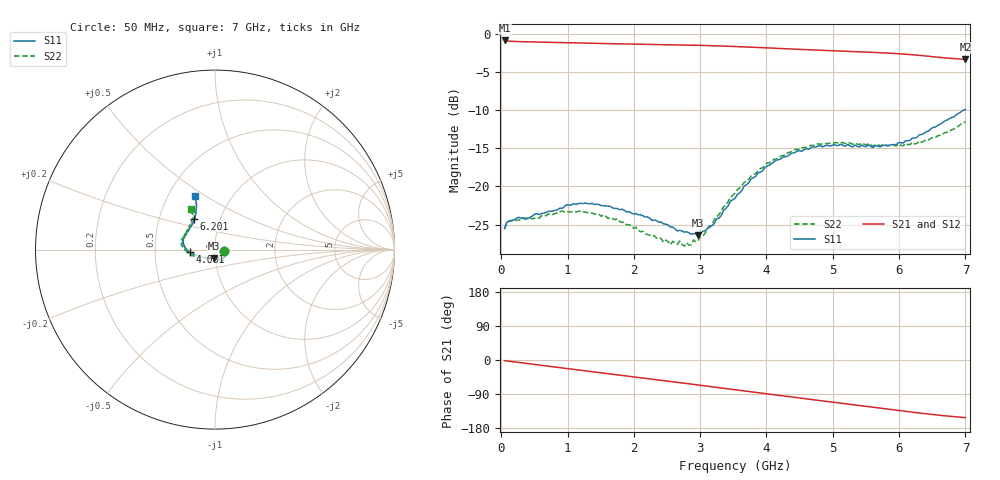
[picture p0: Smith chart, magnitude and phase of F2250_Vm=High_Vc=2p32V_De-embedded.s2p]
! Integrated Device Technology
! Corporate Headquarters
! 6024 Silver Creek Valley Road
! San Jose, CA 95138  USA
! Phone:  1-408-284-8200
! Toll Free:  1-800-223-1366
! Webpage:  http://www.idt.com/
! Timing and RF Division
! 515 Groton Road, Suite 102
! Westford, MA 01886-6024
! Device:  F2250
! Description: Voltage Variable RF Attenuator
! Frequency:  50.0 -  6000.00 MHz
! Package:  3x3 mm Thin QFN Plastic Package: 16 pin
! Ports:  2 RF, 3 DC
!  Pin  1  = GND
!  Pin  2  = NC
!  Pin  3  = RF1  = Port 1
!  Pin  4  = NC
!  Pin  5  = GND
!  Pin  6  = GND
!  Pin  7  = GND
!  Pin  8  = GND
!  Pin  9  = NC
!  Pin 10  = RF2  = Port 2
!  Pin 11  = NC
!  Pin 12  = GND
!  Pin 13  = GND
!  Pin 14  = VCNTRL
!  Pin 15  = VDD
!  Pin 16  = VMODE
! Vcntrl:  2.320 Volts
! Vmode:  +3.300 Volts
! Vdd:  +3.30  Volts
! Current:  1.314 mA
! Data:  The device was measured on a the F2250 evaluation board which has
!  individual transmission lines to the RF pins.  Data was collected
!  using a calibrated network analyzer.  The evaluation board was
!  de-embedded using a TRL calibration technique.
!  The reference plane is the edge of the package pin.
! Misc:  SN 10
!  Action Tracker AT0258
! Date Measured:  2014-11-26
! Date:  2015-10-15  MJV
! Note:
!  Integrated Device Technology supplies this data as a sample of measured
!  data at the package pin for this product.  Your particular data for this
!  product may vary.
!  Data was taken at 25 degrees C.
!  Integrated Device Technology reserves the right to change this data at anytime.
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# GHz S dB R 50
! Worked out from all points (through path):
!   201 points, 50 MHz to 7 GHz, reference 50 ohm
!   highest |S21| = -0.90 dB at 50 MHz (marker M1); lowest = -3.4 dB at 7 GHz (marker M2)
!   group delay of S21, straight-line fit = 61.2 ps
!   lowest |S11| = -26.3 dB at 2.969 GHz (marker M3), VSWR 1.10, Z = 49.2 - j4.73 ohm
!   |S11| at or under -10 dB: start of sweep to 6.978 GHz
!   |S22| runs from -27.8 to -11.5 dB; largest |S21 - S12| = 0.0019
!   S11 on the Smith chart (normalised r, x): 50 MHz: 1.11, -0.02; 4.081 GHz: 0.75, -0.02; 6.201 GHz: 0.75, +0.27; 7 GHz: 0.68, +0.45
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0.05  -25.45 -10.4  -0.90 -1.8  -0.90 -1.8  -25.61 -10.7
0.1195  -24.55 -10.0  -1.00 -3.2  -1.00 -3.2  -24.49 -8.8
0.57125  -23.66 -30.8  -1.11 -13.3  -1.11 -13.3  -24.15 -31.1
0.91875  -22.85 -49.5  -1.18 -21.0  -1.18 -21.1  -23.20 -50.6
1.2315  -22.24 -57.3  -1.25 -27.9  -1.25 -27.9  -23.31 -61.2
1.75275  -22.90 -64.2  -1.34 -39.1  -1.34 -39.1  -24.24 -67.6
2.37825  -24.67 -64.0  -1.43 -52.8  -1.44 -52.8  -26.63 -67.1
2.552  -25.31 -68.7  -1.46 -56.7  -1.46 -56.7  -27.60 -73.6
2.691  -25.73 -76.7  -1.48 -59.8  -1.48 -59.8  -27.13 -81.2
2.7605  -25.97 -78.8  -1.50 -61.3  -1.50 -61.3  -27.80 -85.7
2.969  -26.33 -96.6  -1.54 -66.0  -1.54 -66.0  -27.05 -104.9
3.1775  -25.14 -119.5  -1.59 -70.7  -1.59 -70.7  -25.08 -126.5
3.525  -21.55 -151.9  -1.69 -78.5  -1.69 -78.6  -20.88 -148.5
3.76825  -19.00 -164.1  -1.78 -84.0  -1.79 -84.1  -18.63 -159.5
4.081  -16.99 -175.2  -1.91 -91.0  -1.91 -91.0  -16.68 -171.3
4.4285  -15.57 176.4  -2.04 -98.6  -2.05 -98.7  -15.16 178.8
4.7065  -14.80 169.4  -2.14 -104.8  -2.14 -104.8  -14.66 173.0
5.054  -14.64 161.3  -2.27 -112.5  -2.27 -112.5  -14.25 166.0
5.85325  -14.61 135.4  -2.57 -130.0  -2.57 -130.1  -14.66 147.3
6.20075  -13.66 123.8  -2.78 -137.7  -2.78 -137.8  -14.25 138.3
6.54825  -12.22 115.8  -3.05 -144.7  -3.05 -144.9  -13.58 126.9
7  -9.94 110.9  -3.38 -152.1  -3.39 -152.2  -11.54 120.7
